PROGRAM MAIN_CM
VAR CONSTANT
	cInitIntRMS 	: ST_CM_IntegratedRMS_InitPars   := (	nFFT_Length				:= cFFTLength, 
															nWindowLength			:= cWindowLength,
															fSampleRate 			:= cSampleRate,
		 													fLowerFrequencyLimit	:= cfLowerFrequencyLimit,
															fUpperFrequencyLimit	:= cfUpperFrequencyLimit,
															nMaxBands				:= 1,
															nOrder					:= cOrderRMS,
															nChannels				:= cChannels,                        
															eWindowType				:= cWindowType, 
															nOverlap				:= cOverlap,
															bTransformToDecibel		:= FALSE);	
															
	cInitEmpiricalMom : ST_CM_EmpiricalMoments_InitPars := (nChannels				:= cChannels,
															nSubChannels			:= cOrderRMS + 1);

	cInitClass : ST_CM_DiscreteClassification_InitPars :=(	nChannels				:= cChannels,
															nSubChannels			:= cOrderRMS + 1,
															nMaxClasses				:= cMaxClasses);

END_VAR

VAR	
	fbRMS				: FB_CMA_IntegratedRMS := (stInitPars := cInitIntRMS, nOwnID := eID_IntegratedRMS, aDestIDs := [eID_IntegratedRMS_Sink, eID_EmpiricalMean, eID_EmpiricalStd], nResultBuffers := 5);
	fbMean				: FB_CMA_EmpiricalMean := (stInitPars := cInitEmpiricalMom, nOwnID := eID_EmpiricalMean, aDestIDs := [eID_Classify, eID_EmpiricalMean_Sink]);
	fbStd				: FB_CMA_EmpiricalStandardDeviation := (stInitPars := cInitEmpiricalMom, nOwnID := eID_EmpiricalStd, aDestIDs := [eID_EmpiricalStd_Sink]);
	fbClassification 	: FB_CMA_DiscreteClassification := (stInitPars := cInitClass, nOwnID := eID_Classify, aDestIDS := [eID_Classify_Sink]);													
	
	bConfigureClassification	: BOOL := TRUE;
	aConfigureClassification	: ARRAY[0..cOrderRMS] OF ARRAY[1..cMaxClasses] OF LREAL;
	nClass						: UDINT;
END_VAR

// Configure classification
MAIN_CM.ConfigureClassifications();

// Call IntegratedRMS
fbRMS.Call();
IF fbRMS.bError THEN
	fbErrHist.AddError(bErr:=TRUE, hrErrCode:=fbRMS.hrErrorCode, sErrSource:='MAIN_CM.fbRMS.Call()'); // error monitoring
	// ToDo: if error
END_IF

// Call EmpiricalMean: calculate mean
fbMean.CallEx(nAppendData := cAppendData, bResetData := cResetData);
IF fbMean.bError THEN
	fbErrHist.AddError(bErr:=TRUE, hrErrCode:=fbMean.hrErrorCode, sErrSource:='MAIN_CM.fbMean.CallEx()'); // error monitoring
	// ToDo: if error
END_IF

// Call EmpiricalStd: calculate standard deviation
fbStd.CallEx(nAppendData := cAppendData, bResetData := cResetData);
IF fbStd.bError THEN
	fbErrHist.AddError(bErr:=TRUE, hrErrCode:=fbStd.hrErrorCode, sErrSource:='MAIN_CM.fbStd.CallEx()'); // error monitoring
	// ToDo: if error
END_IF

// Call Classification
fbClassification.Call();
IF fbClassification.bError THEN
	fbErrHist.AddError(bErr := TRUE, hrErrCode := fbClassification.hrErrorCode, sErrSource := 'MAIN_CM.fbClassification.Call()'); // error monitoring
	// ToDo: if error
END_IF

ACTION ConfigureClassifications:
(* configure classification *)
IF bConfigureClassification THEN
	// Copy values
	FOR nClass := 1 TO cMaxClasses DO
		aConfigureClassification[0][nClass] := cISOClassDef_Acc[nClass];		// vibration
		aConfigureClassification[1][nClass] := cISOClassDef_Vel[nClass];		// velocity
		aConfigureClassification[2][nClass] := cISOClassDef_Displ[nClass];		// displacement
	END_FOR

	// Call configure method
	fbClassification.Configure(pArg := ADR(aConfigureClassification), nArgSize := SIZEOF(aConfigureClassification));
	IF NOT fbClassification.bError THEN
		// reset for next configuration
		bConfigureClassification := FALSE;
	ELSE
		fbErrHist.AddError(bErr := TRUE, hrErrCode := fbClassification.hrErrorCode, sErrSource := 'MAIN_CM.fbClassification.Configure()');
	END_IF		
END_IF
END_ACTION

END_PROGRAM
